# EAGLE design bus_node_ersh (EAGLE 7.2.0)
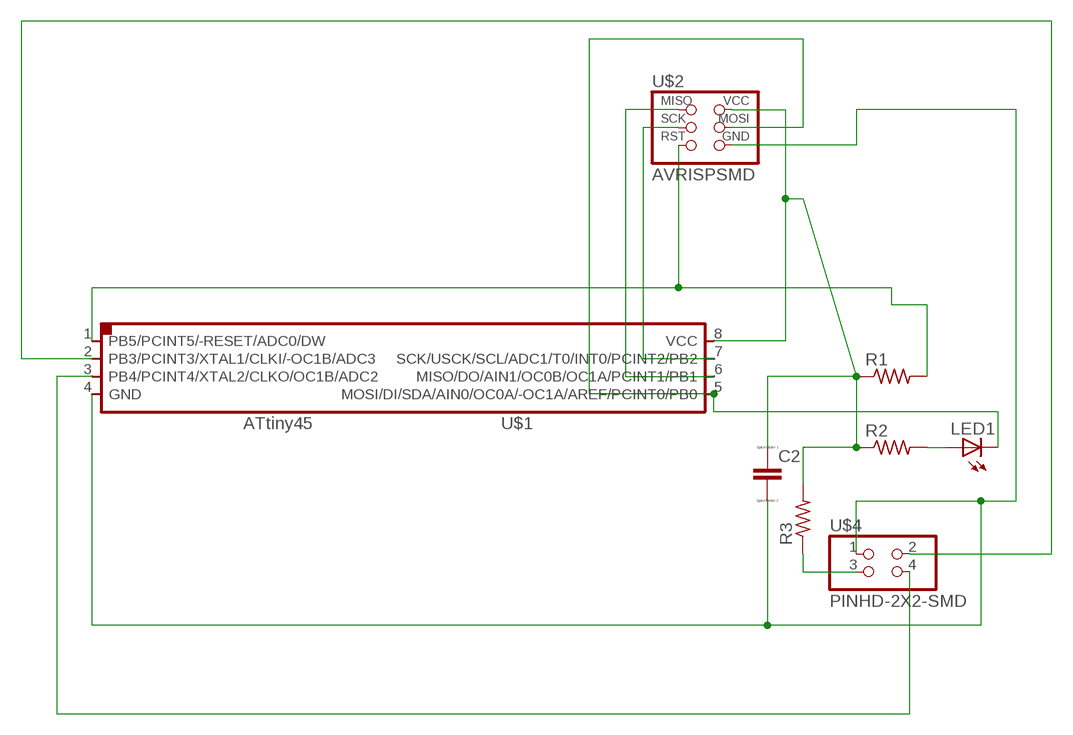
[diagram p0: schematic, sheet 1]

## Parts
C2  CC1206  [C1206]
LED1  LEDKA-3528ASYC  [KA-3528ASYC]
R1  RES-US1206  [R1206]
R2  RES-US1206  [R1206]
R3  RES-US1206  [R1206]
U$1  ATTINY45SI  [SOIC8]
U$2  AVRISPSMD  [2X03SMD]
U$4  PINHD-2X2-SMD  [2X02SMD]

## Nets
N$1: C2.1 R1.1 R2.1 R3.2 U$1.8(VCC) U$2.2(VCC)
N$2: C2.2 U$1.4(GND) U$2.6(GND) U$4.1
N$3: R1.2 U$1.1(PB5/PCINT5/-RESET/ADC0/DW) U$2.5(RST)
N$4: LED1.A R2.2
N$5: LED1.C U$1.5(MOSI/DI/SDA/AIN0/OC0A/-OC1A/AREF/PCINT0/PB0) U$2.4(MOSI)
N$6: U$1.6(MISO/DO/AIN1/OC0B/OC1A/PCINT1/PB1) U$2.1(MISO)
N$7: U$1.7(SCK/USCK/SCL/ADC1/T0/INT0/PCINT2/PB2) U$2.3(SCK)
N$8: U$1.2(PB3/PCINT3/XTAL1/CLKI/-OC1B/ADC3) U$4.2
N$9: U$1.3(PB4/PCINT4/XTAL2/CLKO/OC1B/ADC2) U$4.4
N$10: R3.1 U$4.3

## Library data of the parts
C2 = eagle-ltspice:C: CAPACITOR, European symbol; SPICEMODEL: NONE; SPICEPREFIX: C
LED1 = led:LED: LED
R1-R3 = fab:RES-US: Resistor (US Symbol)
U$1 = fab:ATTINY45
U$2 = fab:AVRISP
U$4 = fab:PINHD-2X2-SMD

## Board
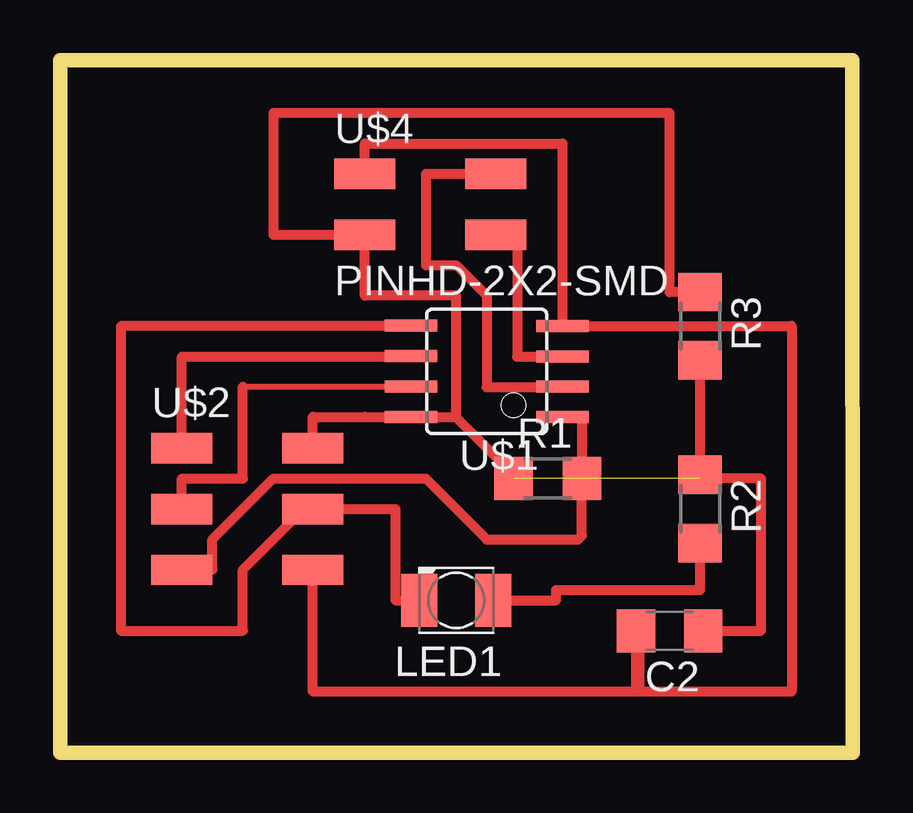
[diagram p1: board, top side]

Size 33.04 x 28.88 mm. Coordinates in mm from the lower left corner, seen from the top.
Outline: 0,0 33.04,0 33,28.88 0,28.88 0,0
Copper layers (1*16): Top 0.035mm / dielectric 1.5mm / Bottom 0.035mm
Design rules "default": minimum track width 10mil, minimum drill 24mil, track to track 8mil, track to pad 8mil, pad to pad 8mil, via to via 8mil, smd to smd 8mil, copper to edge 40mil, drill to drill 8mil, minimum pad ring 10mil, minimum via ring 8mil, stop-mask expansion 4mil, vias tented up to drill 0mil, thermal gap 10mil

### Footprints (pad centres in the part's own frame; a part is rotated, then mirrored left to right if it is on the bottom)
C1206 = smd 1.6 x 1.8: 1 -1.4,0; 2 1.4,0
KA-3528ASYC = smd 1.5 x 2.2: A -1.55,0; C 1.55,0
R1206 = smd 1.6 x 1.803: 1 -1.422,0; 2 1.422,0
SOIC8 = smd 0.5 x 2.2: 1 -1.905,-3.154; 2 -0.645,-3.154; 3 0.625,-3.154; 4 1.895,-3.154; 5 1.905,3.154; 6 0.635,3.154; 7 -0.635,3.154; 8 -1.905,3.154
2X03SMD = smd 2.54 x 1.27: 1 -2.54,2.54; 2 2.92,2.54; 3 -2.54,0; 4 2.92,0; 5 -2.54,-2.54; 6 2.92,-2.54
2X02SMD = smd 2.54 x 1.27: 1 -2.54,1.27; 2 2.92,1.27; 3 -2.54,-1.27; 4 2.92,-1.27

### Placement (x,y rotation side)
C2  25.4,5.08 180 top
LED1  16.51,6.35 180 top
R1  20.32,11.43 0 top
R2  26.67,10.16 270 top
R3  26.67,17.78 270 top
U$1  17.78,15.9 90 top
U$2  7.62,10.16 0 top
U$4  15.24,22.86 0 top

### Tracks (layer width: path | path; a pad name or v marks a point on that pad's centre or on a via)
N$1  (1 unrouted)
  Top 0.254: 12.7,14 U$1.8
  Top 0.406: U$2.2 10.54,14 12.7,14 16.49,14 16.51,13.97 | C2.1 29.21,5.08 29.21,11.43 26.67,11.43 R2.1 R3.2 | R1.1 18.9,11.58 16.51,13.97 | 16.51,13.97 16.51,19.05 12.7,19.05 12.7,21.59
N$2
  Top 0.406: U$4.1 12.7,25.4 20.93,25.4 U$1.4 30.48,17.79 30.48,2.54 24.13,2.54 | 24.13,2.54 24,2.54 | 24,2.54 C2.2 24.13,5.08 24.13,2.54 | 24,2.54 10.54,2.54 U$2.6
N$3
  Top 0.406: U$2.5 6.35,7.62 6.35,8.89 8.89,11.43 15.24,11.43 17.78,8.89 21.59,8.89 21.74,9.04 R1.2 21.74,14 U$1.1
N$4
  Top 0.406: LED1.A 20.68,6.35 20.68,6.78 26.67,6.78 R2.2
N$5
  Top 0.254: U$1.5 14.63,17.78 | 10.16,10.16 U$2.4 | 15.24,6.35 LED1.C
  Top 0.406: 14.63,17.78 2.54,17.78 2.54,5.08 7.62,5.08 7.62,7.62 10.16,10.16 | U$2.4 13.97,10.16 13.97,6.35 LED1.C
N$6
  Top 0.254: 14.63,16.51 U$1.6
  Top 0.406: U$2.1 5.08,16.51 14.63,16.51
N$7
  Top 0.254: 7.62,15.27 U$1.7
  Top 0.406: U$2.3 5.08,11.43 7.62,11.43 7.62,15.27
N$8
  Top 0.254: 20.93,15.24 U$1.2
  Top 0.406: U$4.2 15.24,24.13 15.24,20.32 16.51,20.32 17.78,19.05 17.78,15.24 20.93,15.24
N$9
  Top 0.406: U$4.4 19.05,21.59 19.05,16.51 20.93,16.51 U$1.3
N$10
  Top 0.406: R3.1 25.4,19.2 25.4,26.67 8.89,26.67 8.89,21.59 U$4.3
